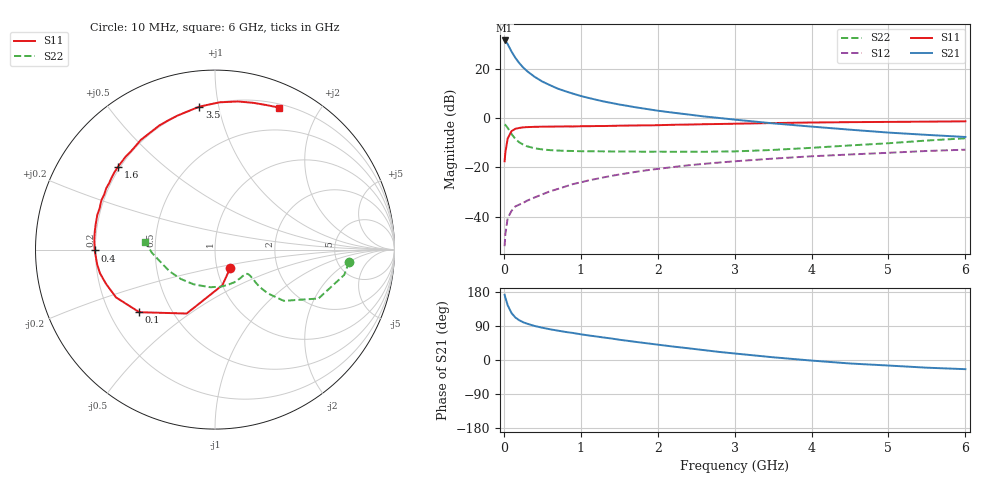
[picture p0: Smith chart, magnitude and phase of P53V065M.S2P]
! SIEMENS Small Signal Semiconductors
! BFP183
! Si NPN RF Bipolar Junction Transistor in SOT143
! VCE = 3 V  IC = 65 mA
! Common Emitter S-Parameters:  March  1996
# GHz  S  MA  R  50
!  f  S11  S21  S12  S22
! GHz  MAG  ANG  MAG  ANG  MAG  ANG  MAG  ANG
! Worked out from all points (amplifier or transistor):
!   36 points, 10 MHz to 6 GHz, reference 50 ohm
!   highest |S21| = 31.7 dB at 10 MHz (marker M1)
!   |S21| within 3 dB of that: start of sweep to 74.82 MHz
!   unconditionally stable (mu >= 1): start of sweep to 31.91 MHz; 184.4 MHz to end of sweep
!   at 250 MHz: K = 1.18, MAG = 25.0 dB, |S12| = -34.5 dB
!   at 1.4 GHz: K = 1.69, MAG = 10.0 dB, |S12| = -23.4 dB
!   at 6 GHz: K = 1.27, MAG = -0.5 dB, |S12| = -12.8 dB
!   S11 on the Smith chart (normalised r, x): 10 MHz: 1.16, -0.25; 100 MHz: 0.33, -0.33; 400 MHz: 0.20, -0.00; 1.6 GHz: 0.19, +0.36; 3.5 GHz: 0.20, +0.88; 6 GHz: 0.24, +1.52
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0.01  0.1339 -51.1  38.39 172.2  0.0025 60.9  0.7505 -5.2
0.02  0.2023 -78.2  37.51 164.6  0.0044 63.3  0.7334 -11.1
0.05  0.3896 -113.9  32.26 144.5  0.0093 62.6  0.6378 -25.3
0.1  0.5473 -140.4  22.84 123.8  0.0131 49.7  0.4778 -36.7
0.15  0.6123 -154.2  16.99 112.1  0.0161 46.7  0.3809 -39.7
0.2  0.6363 -162.5  13.32 104.9  0.0175 48.0  0.3248 -39.9
0.25  0.6543 -168.4  10.88 99.7  0.0189 49.6  0.2926 -39.0
0.3  0.6614 -172.6  9.177 96.0  0.021 52.6  0.2701 -37.9
0.4  0.6704 -179.6  6.98 89.8  0.0245 54.9  0.2457 -36.7
0.5  0.6749 175.3  5.603 85.2  0.0283 57.4  0.2325 -36.4
0.6  0.6777 170.9  4.723 81.1  0.0327 59.5  0.2251 -36.9
0.7  0.6802 167.1  4.022 77.6  0.0364 61.0  0.2205 -37.8
0.9  0.6826 160.4  3.17 71.3  0.0459 62.0  0.2159 -41.1
1.1  0.6897 153.3  2.602 64.8  0.0544 61.7  0.2128 -45.2
1.3  0.6962 147.9  2.198 59.3  0.0629 61.3  0.2122 -50.0
1.6  0.711 139.4  1.8 50.9  0.0761 59.5  0.2114 -57.6
2.2  0.7381 124.0  1.302 35.5  0.1019 54.1  0.208 -76.0
2.8  0.766 109.7  1.015 21.3  0.1259 47.9  0.2112 -96.7
3.5  0.8014 96.2  0.789 7.2  0.1513 41.0  0.2273 -121.9
4.5  0.835 81.2  0.587 -9.2  0.1835 30.6  0.2806 -154.4
5.5  0.855 70.3  0.46 -20.3  0.2164 21.3  0.353 -177.3
6  0.8679 65.7  0.417 -24.2  0.2299 16.0  0.3916 173.4
